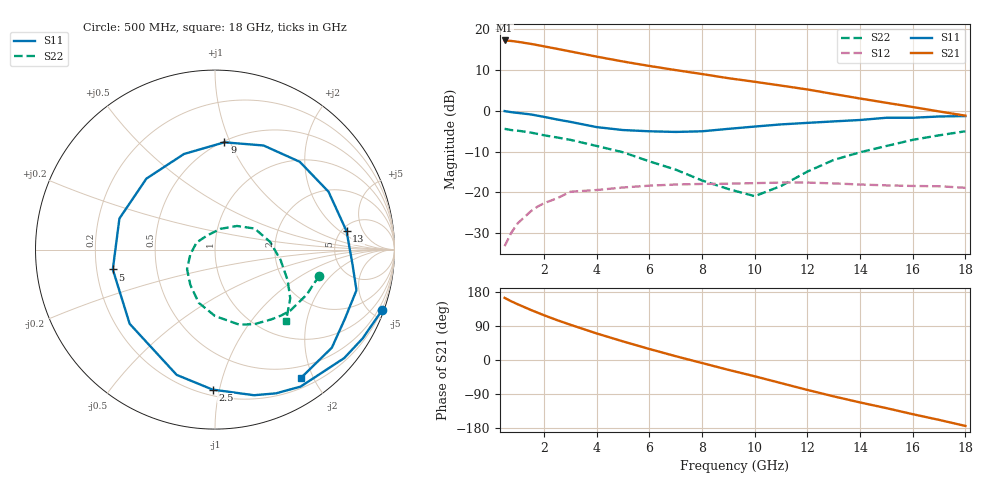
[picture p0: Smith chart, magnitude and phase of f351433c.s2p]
!ATF-35143
!S-PARAMETERS at Vds=3V  Id=15mA.  LAST UPDATED 06-3-99
# ghz s ma r 50
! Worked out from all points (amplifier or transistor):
!   23 points, 500 MHz to 18 GHz, reference 50 ohm
!   highest |S21| = 17.2 dB at 500 MHz (marker M1)
!   |S21| within 3 dB of that: start of sweep to 3.243 GHz
!   unconditionally stable (mu >= 1): 7.514 GHz to end of sweep
!   at 1.5 GHz: K = 0.26, MSG = 20.5 dB, |S12| = -24.6 dB
!   at 7 GHz: K = 0.95, MSG = 14.0 dB, |S12| = -18.1 dB
!   at 18 GHz: K = 1.34, MAG = 5.4 dB, |S12| = -18.9 dB
!   lowest NFmin = 0.11 dB at 500 MHz
!   S11 on the Smith chart (normalised r, x): 500 MHz: 0.17, -5.67; 2.5 GHz: 0.24, -0.95; 5 GHz: 0.27, -0.09; 9 GHz: 0.51, +0.95; 13 GHz: 5.52, +2.51; 18 GHz: 0.33, -1.83
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0.5  0.99 -20.0  7.24 164.0  0.022 77.0  0.6 -14.0
0.75  0.96 -31.0  7.14 155.0  0.032 70.0  0.58 -20.0
1  0.94 -40.0  6.97 147.0  0.042 65.0  0.57 -26.0
1.5  0.9 -58.0  6.57 132.0  0.059 54.0  0.54 -39.0
1.75  0.87 -67.0  6.35 125.0  0.067 49.0  0.52 -45.0
2  0.84 -75.0  6.13 118.0  0.074 44.0  0.5 -51.0
2.5  0.78 -91.0  5.71 105.0  0.085 35.0  0.47 -62.0
3  0.73 -107.0  5.31 93.0  0.102 27.0  0.44 -72.0
4  0.63 -139.0  4.59 70.0  0.107 11.0  0.37 -90.0
5  0.58 -169.0  4 49.0  0.115 -2.0  0.31 -107.0
6  0.56 162.0  3.53 29.0  0.121 -15.0  0.24 -125.0
7  0.55 134.0  3.14 10.0  0.125 -28.0  0.19 -145.0
8  0.56 108.0  2.81 -8.0  0.127 -39.0  0.14 -169.0
9  0.6 85.0  2.5 -26.0  0.128 -50.0  0.11 159.0
10  0.64 65.0  2.26 -43.0  0.13 -61.0  0.09 119.0
11  0.68 46.0  2.03 -61.0  0.132 -71.0  0.12 75.0
12  0.71 27.0  1.82 -79.0  0.132 -83.0  0.18 47.0
13  0.74 8.0  1.6 -96.0  0.129 -94.0  0.25 28.0
14  0.77 -6.0  1.41 -112.0  0.125 -104.0  0.31 8.0
16  0.82 -28.0  1.11 -143.0  0.12 -123.0  0.44 -23.0
17  0.85 -40.0  0.98 -158.0  0.119 -134.0  0.5 -33.0
18  0.86 -56.0  0.87 -174.0  0.114 -144.0  0.56 -45.0
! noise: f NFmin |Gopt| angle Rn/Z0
0.5  0.11  0.86  4  0.17
0.9  0.15  0.81  12  0.16
1.5  0.21  0.73  25  0.15
1.8  0.24  0.69  32  0.14
2.5  0.31  0.6  47  0.17
3  0.37  0.55  59  0.15
5  0.58  0.4  115  0.07
6  0.68  0.36  147  0.05
8  0.89  0.32  -146  0.07
10  1.1  0.33  -77  0.22
